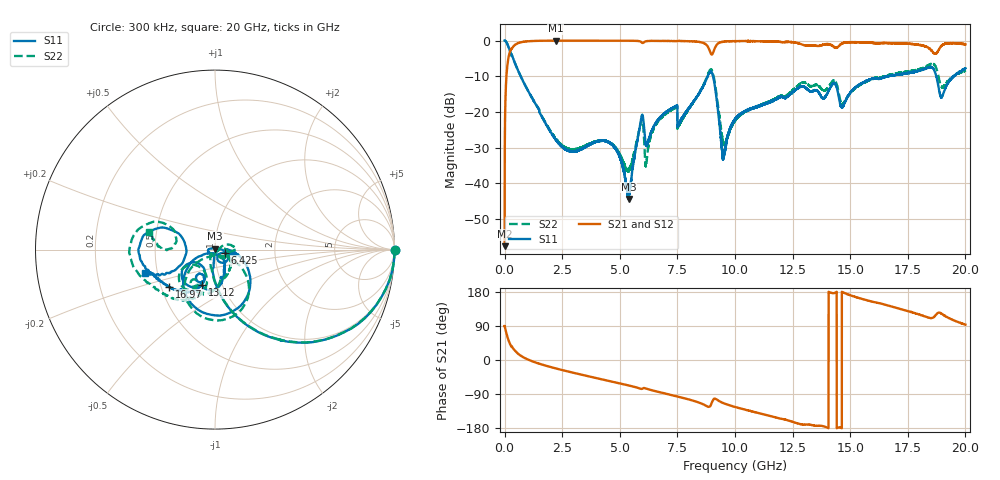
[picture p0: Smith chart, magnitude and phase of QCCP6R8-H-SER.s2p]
!QCCP6R8
!Johanson Technology Inc.
!www.johansontechnology.com
!Test Board Conditions:
!Substrate Type  RO4350B
!Substrate Thickness  20 mil
!Substrate Dk  3.66
!TL Type: GCPW
!TL Trace Width  36 mil
!TL Gap  12 mil
!Electrode orientation  Horizontal
!DUT TOPOLOGY	SERIES
!Mounting Pad LxW  26x36 mil
# MHz S  dB  R 50
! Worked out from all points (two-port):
!   20001 points, 300 kHz to 20 GHz, reference 50 ohm
!   highest |S21| = -0.03 dB at 2.21 GHz (marker M1); lowest = -57.6 dB at 300 kHz (marker M2)
!   |S21| within 3 dB of the highest: 238.9 MHz to 8.914 GHz (8.675 GHz wide, 190 % of centre); 9.073 GHz to 18.56 GHz (9.492 GHz wide, 68.7 % of centre)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
!   lowest |S11| = -44.3 dB at 5.388 GHz (marker M3), VSWR 1.01, Z = 50.1 + j0.595 ohm
!   |S11| at or under -10 dB: 698.3 MHz to 8.815 GHz (8.117 GHz wide, 171 % of centre); 9.047 GHz to 16.62 GHz (7.574 GHz wide, 59 % of centre); 18.74 GHz to 19.49 GHz (749.6 MHz wide, 3.92 % of centre)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
!   |S22| runs from -36.8 to 0.0 dB; largest |S21 - S12| = 0.041
!   S11 on the Smith chart (normalised r, x): 300 kHz: open; 6.425 GHz: 1.11, -0.04; 13.12 GHz: 0.80, -0.33; 16.97 GHz: 0.55, -0.26; 20 GHz: 0.43, -0.13
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0.3  0.00 -0.2  -57.55 89.5  -58.00 86.7  0.02 -0.0
108.298  -0.81 -25.6  -7.67 64.1  -7.70 64.2  -0.82 -25.7
258.296  -3.45 -50.1  -2.70 39.4  -2.69 39.4  -3.46 -50.0
2210.267  -27.70 -95.9  -0.03 -22.0  -0.04 -22.0  -27.42 -125.4
3334.25  -30.42 -131.7  -0.04 -38.7  -0.04 -38.7  -29.94 -124.2
4636.23  -28.97 177.1  -0.05 -56.8  -0.06 -56.8  -28.92 -103.8
5388.219  -44.34 78.3  -0.07 -67.3  -0.06 -67.3  -36.75 -37.1
5924.211  -21.91 -24.2  -0.40 -76.2  -0.41 -76.3  -22.62 -9.6
6158.208  -29.54 -49.0  -0.18 -75.8  -0.20 -75.8  -34.12 3.4
6425.204  -24.75 -19.2  -0.10 -80.3  -0.10 -80.3  -25.39 26.4
6667.2  -22.14 -17.6  -0.09 -84.1  -0.12 -84.1  -22.59 22.8
7600.186  -22.81 -0.7  -0.12 -97.9  -0.12 -97.9  -23.36 -27.8
8943.166  -8.68 -85.4  -3.52 -120.2  -3.53 -120.0  -8.07 -83.9
9488.158  -32.78 -103.6  -0.32 -113.4  -0.33 -113.6  -28.52 -107.5
10000.15  -21.98 -50.3  -0.15 -123.9  -0.17 -123.9  -22.54 -33.1
13115.1  -13.51 -110.2  -1.43 -170.4  -1.46 -170.5  -12.10 -115.8
13334.1  -14.21 -112.2  -1.33 -171.6  -1.34 -171.7  -12.79 -117.8
16667.05  -10.00 -136.3  -0.72 143.3  -0.66 142.6  -9.66 -121.1
16966.05  -9.64 -141.0  -0.79 138.3  -0.72 137.7  -9.22 -126.1
18529.02  -7.49 177.7  -2.80 110.7  -2.98 110.2  -6.46 -174.7
18971.01  -15.90 -174.4  -1.45 122.1  -1.49 122.5  -13.00 164.5
20000  -7.74 -161.6  -1.04 93.3  -0.88 94.9  -8.38 164.6
